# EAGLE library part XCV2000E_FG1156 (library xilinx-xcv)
xcv2000e_fg1156 edit this description Auto generated by make-symbol-device-package-bsdl.ulp Rev. 26 Source: xcv2000e_fg1156.bsd
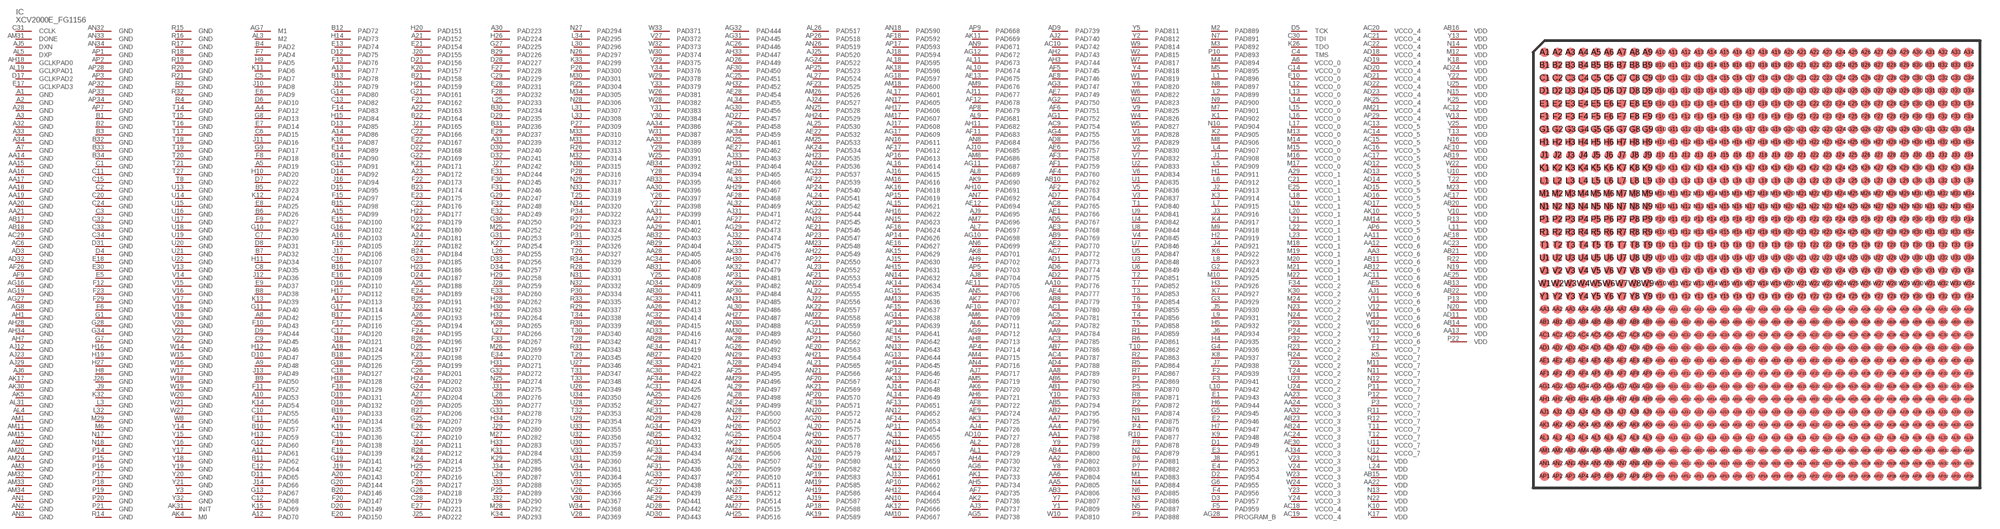
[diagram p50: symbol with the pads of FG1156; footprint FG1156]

Designator prefix IC

## XCV2000E_FG1156 (OC_FARNELL: unknown; OC_NEWARK: unknown)  [FG1156]
A1  GND  pwr
A2  GND  pwr
A3  GND  pwr
A4  PAD12
A5  PAD19
A6  VCCO_0  pwr
A7  GND  pwr
A8  PAD42
A9  PAD48
A10  PAD53
A11  PAD61
A12  PAD70
A13  PAD77
A14  PAD86
A15  PAD99
A16  PAD103
A17  PAD113
A18  PAD124
A19  PAD134
A20  PAD143
A21  PAD152
A22  PAD163
A23  PAD172
A24  PAD181
A25  PAD188
A26  PAD193
A27  PAD204
A28  GND  pwr
A29  VCCO_1  pwr
A30  PAD223
A31  PAD239
A32  GND  pwr
A33  GND  pwr
A34  GND  pwr
AA1  PAD798
AA2  PAD802
AA3  VCCO_6  pwr
AA4  PAD797
AA5  PAD805
AA6  PAD804
AA7  PAD796
AA8  PAD789
AA9  PAD784
AA10  PAD776
AA11  VCCO_6  pwr
AA12  VCCO_6  pwr
AA13  VDD  pwr
AA14  GND  pwr
AA15  GND  pwr
AA16  GND  pwr
AA17  GND  pwr
AA18  GND  pwr
AA19  GND  pwr
AA20  GND  pwr
AA21  GND  pwr
AA22  VDD  pwr
AA23  VCCO_3  pwr
AA24  VCCO_3  pwr
AA25  PAD426
AA26  PAD413
AA27  PAD401
AA28  PAD405
AA29  PAD402
AA30  PAD396
AA31  PAD399
AA32  VCCO_3  pwr
AA33  PAD389
AA34  PAD386
AB1  PAD792
AB2  PAD795
AB3  PAD806
AB4  PAD800
AB5  PAD794
AB6  PAD790
AB7  PAD786
AB8  PAD779
AB9  PAD769
AB10  PAD762
AB11  VCCO_6  pwr
AB12  VCCO_6  pwr
AB13  VDD  pwr
AB14  VDD  pwr
AB15  VDD  pwr
AB16  VDD  pwr
AB17  GND  pwr
AB18  GND  pwr
AB19  VDD  pwr
AB20  VDD  pwr
AB21  VDD  pwr
AB22  VDD  pwr
AB23  VCCO_3  pwr
AB24  VCCO_3  pwr
AB25  PAD432
AB26  PAD415
AB27  PAD420
AB28  PAD417
AB29  PAD404
AB30  PAD411
AB31  PAD407
AB32  PAD403
AB33  PAD395
AB34  PAD392
AC1  PAD780
AC2  PAD782
AC3  PAD785
AC4  PAD787
AC5  PAD781
AC6  GND  pwr
AC7  PAD772
AC8  PAD765
AC9  PAD754
AC10  PAD742
AC11  VCCO_6  pwr
AC12  VDD  pwr
AC13  VCCO_5  pwr
AC14  VCCO_5  pwr
AC15  VCCO_5  pwr
AC16  VCCO_5  pwr
AC17  VCCO_5  pwr
AC18  VCCO_4  pwr
AC19  VCCO_4  pwr
AC20  VCCO_4  pwr
AC21  VCCO_4  pwr
AC22  VCCO_4  pwr
AC23  VDD  pwr
AC24  VCCO_3  pwr
AC25  PAD451
AC26  PAD446
AC27  PAD438
AC28  PAD435
AC29  GND  pwr
AC30  PAD422
AC31  PAD425
AC32  PAD414
AC33  PAD412
AC34  PAD406
AD1  PAD773
AD2  PAD775
AD3  GND  pwr
AD4  PAD788
AD5  PAD767
AD6  PAD774
AD7  PAD764
AD8  PAD756
AD9  PAD739
AD10  PAD727
AD11  VDD  pwr
AD12  VCCO_5  pwr
AD13  VCCO_5  pwr
AD14  VCCO_5  pwr
AD15  VCCO_5  pwr
AD16  VCCO_5  pwr
AD17  VCCO_5  pwr
AD18  VCCO_4  pwr
AD19  VCCO_4  pwr
AD20  VCCO_4  pwr
AD21  VCCO_4  pwr
AD22  VCCO_4  pwr
AD23  VCCO_4  pwr
AD24  VDD  pwr
AD25  PAD461
AD26  PAD449
AD27  PAD457
AD28  PAD442
AD29  PAD429
AD30  PAD443
AD31  PAD433
AD32  GND  pwr
AD33  PAD416
AD34  PAD409
AE1  PAD766
AE2  PAD770
AE3  PAD768
AE4  PAD777
AE5  VCCO_6  pwr
AE6  PAD757
AE7  PAD749
AE8  PAD746
AE9  PAD724
AE10  VDD  pwr
AE11  PAD705
AE12  PAD694
AE13  PAD675
AE14  PAD641
AE15  PAD642
AE16  PAD627
AE17  VDD  pwr
AE18  VDD  pwr
AE19  PAD571
AE20  PAD563
AE21  PAD546
AE22  PAD532
AE23  PAD514
AE24  PAD499
AE25  VDD  pwr
AE26  PAD465
AE27  PAD462
AE28  PAD454
AE29  PAD441
AE30  VCCO_3  pwr
AE31  PAD428
AE32  PAD427
AE33  PAD421
AE34  PAD419
AF1  PAD759
AF2  PAD763
AF3  PAD758
AF4  PAD760
AF5  PAD745
AF6  PAD751
AF7  PAD735
AF8  PAD722
AF9  GND  pwr
AF10  PAD708
AF11  PAD683
AF12  PAD678
AF13  PAD651
AF14  PAD653
AF15  PAD637
AF16  PAD624
AF17  PAD612
AF18  PAD592
AF19  PAD582
AF20  PAD567
AF21  PAD553
AF22  PAD539
AF23  PAD525
AF24  PAD507
AF25  PAD495
AF26  GND  pwr
AF27  PAD472
AF28  PAD468
AF29  PAD458
AF30  PAD450
AF31  PAD436
AF32  PAD439
AF33  PAD434
AF34  PAD424
AG1  PAD752
AG2  PAD750
AG3  PAD747
AG4  PAD755
AG5  PAD738
AG6  PAD732
AG7  M1  in
AG8  GND  pwr
AG9  PAD712
AG10  PAD698
AG11  PAD687
AG12  PAD672
AG13  PAD644
AG14  PAD638
AG15  PAD635
AG16  GND  pwr
AG17  PAD609
AG18  PAD597
AG19  GND  pwr
AG20  PAD574
AG21  PAD559
AG22  PAD544
AG23  PAD537
AG24  PAD522
AG25  PAD504
AG26  PAD492
AG27  GND  pwr
AG28  PROGRAM_B  in
AG29  PAD473
AG30  PAD456
AG31  PAD445
AG32  PAD444
AG33  PAD437
AG34  PAD431
AH1  GND  pwr
AH2  PAD743
AH3  PAD744
AH4  PAD730
AH5  PAD734
AH6  PAD721
AH7  GND  pwr
AH8  PAD713
AH9  PAD702
AH10  PAD691
AH11  PAD682
AH12  PAD664
AH13  PAD657
AH14  PAD645
AH15  PAD631
AH16  PAD622
AH17  PAD606
AH18  GCLKPAD0  in
AH19  PAD586
AH20  PAD577
AH21  PAD564
AH22  PAD549
AH23  PAD535
AH24  PAD529
AH25  PAD516
AH26  PAD503
AH27  PAD487
AH28  GND  pwr
AH29  PAD467
AH30  PAD477
AH31  PAD464
AH32  PAD452
AH33  PAD447
AH34  GND  pwr
AJ1  VCCO_6  pwr
AJ2  PAD740
AJ3  PAD737
AJ4  PAD726
AJ5  DXN  pas
AJ6  GND  pwr
AJ7  PAD717
AJ8  PAD704
AJ9  PAD695
AJ10  PAD685
AJ11  PAD677
AJ12  GND  pwr
AJ13  PAD661
AJ14  PAD648
AJ15  PAD630
AJ16  PAD615
AJ17  PAD608
AJ18  PAD594
AJ19  PAD587
AJ20  PAD580
AJ21  PAD560
AJ22  PAD556
AJ23  GND  pwr
AJ24  PAD527
AJ25  PAD520
AJ26  PAD509
AJ27  PAD502
AJ28  PAD494
AJ29  GND  pwr
AJ30  PAD475
AJ31  PAD471
AJ32  PAD474
AJ33  PAD463
AJ34  VCCO_3  pwr
AK1  PAD733
AK2  PAD736
AK3  PAD725
AK4  M0  in
AK5  GND  pwr
AK6  PAD720
AK7  PAD707
AK8  PAD701
AK9  PAD690
AK10  VCCO_5  pwr
AK11  PAD669
AK12  PAD666
AK13  PAD647
AK14  PAD634
AK15  PAD629
AK16  PAD618
AK17  GND  pwr
AK18  PAD596
AK19  PAD589
AK20  PAD578
AK21  PAD569
AK22  PAD557
AK23  PAD542
AK24  PAD534
AK25  VCCO_4  pwr
AK26  PAD511
AK27  PAD505
AK28  PAD490
AK29  PAD482
AK30  GND  pwr
AK31  INIT
AK32  PAD479
AK33  PAD476
AK34  PAD459
AL1  PAD729
AL2  PAD728
AL3  M2  in
AL4  GND  pwr
AL5  DXP  pas
AL6  PAD711
AL7  PAD697
AL8  PAD689
AL9  PAD681
AL10  PAD674
AL11  PAD673
AL12  PAD660
AL13  PAD655
AL14  PAD649
AL15  PAD621
AL16  PAD614
AL17  PAD601
AL18  PAD595
AL19  GCLKPAD1  in
AL20  PAD575
AL21  PAD565
AL22  PAD555
AL23  PAD552
AL24  PAD541
AL25  PAD530
AL26  PAD517
AL27  PAD524
AL28  PAD498
AL29  PAD497
AL30  PAD486
AL31  GND  pwr
AL32  PAD469
AL33  PAD466
AL34  PAD455
AM1  GND  pwr
AM2  GND  pwr
AM3  GND  pwr
AM4  PAD715
AM5  PAD719
AM6  PAD709
AM7  PAD696
AM8  PAD686
AM9  PAD676
AM10  PAD667
AM11  GND  pwr
AM12  PAD659
AM13  PAD636
AM14  VCCO_5  pwr
AM15  GND  pwr
AM16  PAD616
AM17  PAD607
AM18  PAD600
AM19  PAD585
AM20  GND  pwr
AM21  VCCO_4  pwr
AM22  PAD558
AM23  PAD548
AM24  GND  pwr
AM25  PAD533
AM26  PAD526
AM27  PAD515
AM28  PAD506
AM29  PAD496
AM30  PAD489
AM31  DONE
AM32  GND  pwr
AM33  GND  pwr
AM34  GND  pwr
AN1  GND  pwr
AN2  GND  pwr
AN3  GND  pwr
AN4  PAD716
AN5  PAD706
AN6  PAD699
AN7  PAD692
AN8  PAD684
AN9  PAD671
AN10  PAD665
AN11  PAD656
AN12  PAD652
AN13  PAD643
AN14  PAD632
AN15  PAD623
AN16  PAD611
AN17  PAD605
AN18  PAD590
AN19  PAD579
AN20  PAD572
AN21  PAD566
AN22  PAD554
AN23  PAD545
AN24  PAD536
AN25  PAD528
AN26  PAD519
AN27  PAD512
AN28  PAD500
AN29  PAD493
AN30  PAD488
AN31  PAD485
AN32  GND  pwr
AN33  GND  pwr
AN34  GND  pwr
AP1  GND  pwr
AP2  GND  pwr
AP3  GND  pwr
AP4  PAD714
AP5  PAD703
AP6  VCCO_5  pwr
AP7  GND  pwr
AP8  PAD679
AP9  PAD668
AP10  PAD662
AP11  PAD654
AP12  PAD646
AP13  PAD639
AP14  PAD626
AP15  PAD619
AP16  PAD613
AP17  PAD593
AP18  PAD588
AP19  PAD583
AP20  PAD570
AP21  PAD562
AP22  PAD550
AP23  PAD547
AP24  PAD540
AP25  PAD523
AP26  PAD518
AP27  PAD510
AP28  GND  pwr
AP29  VCCO_4  pwr
AP30  PAD484
AP31  PAD481
AP32  GND  pwr
AP33  GND  pwr
AP34  GND  pwr
B1  GND  pwr
B2  GND  pwr
B3  GND  pwr
B4  PAD2
B5  PAD23
B6  PAD26
B7  PAD32
B8  PAD38
B9  PAD50
B10  PAD57
B11  PAD62
B12  PAD72
B13  PAD78
B14  PAD90
B15  PAD98
B16  PAD108
B17  PAD115
B18  PAD125
B19  PAD133
B20  PAD146
B21  PAD158
B22  PAD164
B23  PAD174
B24  PAD184
B25  PAD191
B26  PAD196
B27  PAD206
B28  PAD212
B29  PAD226
B30  PAD234
B31  PAD236
B32  GND  pwr
B33  GND  pwr
B34  GND  pwr
C1  GND  pwr
C2  GND  pwr
C3  GND  pwr
C4  TMS  in
C5  PAD7
C6  PAD15
C7  PAD30
C8  PAD35
C9  PAD45
C10  PAD55
C11  GND  pwr
C12  PAD68
C13  PAD82
C14  VCCO_0  pwr
C15  GND  pwr
C16  PAD107
C17  PAD120
C18  PAD127
C19  PAD136
C20  GND  pwr
C21  VCCO_1  pwr
C22  PAD166
C23  PAD176
C24  GND  pwr
C25  PAD194
C26  PAD201
C27  PAD210
C28  PAD219
C29  PAD229
C30  TDI  in
C31  CCLK
C32  GND  pwr
C33  GND  pwr
C34  GND  pwr
D1  PAD949
D2  PAD954
D3  PAD957
D4  GND  pwr
D5  TCK  in
D6  PAD10
D7  PAD22
D8  PAD31
D9  PAD44
D10  PAD47
D11  PAD65
D12  PAD75
D13  PAD85
D14  PAD92
D15  PAD95
D16  PAD110
D17  GCLKPAD2  in
D18  PAD132
D19  PAD131
D20  PAD149
D21  PAD156
D22  PAD168
D23  PAD179
D24  PAD187
D25  PAD197
D26  PAD205
D27  PAD216
D28  PAD227
D29  PAD235
D30  PAD240
D31  GND  pwr
D32  PAD241
D33  PAD256
D34  PAD257
E1  PAD943
E2  PAD946
E3  PAD951
E4  PAD953
E5  GND  pwr
E6  PAD9
E7  PAD14
E8  PAD25
E9  PAD37
E10  VCCO_0  pwr
E11  PAD56
E12  PAD64
E13  PAD74
E14  PAD89
E15  PAD100
E16  PAD109
E17  GCLKPAD3  in
E18  GND  pwr
E19  PAD139
E20  PAD150
E21  PAD154
E22  PAD167
E23  PAD175
E24  PAD189
E25  VCCO_1  pwr
E26  PAD209
E27  PAD221
E28  PAD231
E29  PAD237
E30  GND  pwr
E31  PAD244
E32  PAD249
E33  PAD260
E34  PAD270
F1  VCCO_7  pwr
F2  PAD939
F3  PAD941
F4  PAD956
F5  PAD959
F6  GND  pwr
F7  PAD4
F8  PAD18
F9  PAD27
F10  PAD43
F11  PAD52
F12  GND  pwr
F13  PAD76
F14  PAD83
F15  PAD97
F16  PAD105
F17  PAD116
F18  PAD129
F19  PAD138
F20  PAD147
F21  PAD162
F22  PAD173
F23  GND  pwr
F24  PAD195
F25  PAD199
F26  PAD217
F27  PAD228
F28  PAD232
F29  GND  pwr
F30  PAD245
F31  PAD246
F32  PAD248
F33  PAD267
F34  VCCO_2  pwr
G1  GND  pwr
G2  PAD924
G3  PAD929
G4  PAD936
G5  PAD945
G6  PAD955
G7  GND  pwr
G8  PAD13
G9  PAD17
G10  PAD29
G11  PAD40
G12  PAD60
G13  PAD67
G14  PAD80
G15  PAD91
G16  PAD102
G17  PAD114
G18  PAD126
G19  PAD141
G20  PAD144
G21  PAD161
G22  PAD169
G23  PAD185
G24  PAD203
G25  PAD207
G26  PAD218
G27  PAD225
G28  GND  pwr
G29  PAD247
G30  PAD250
G31  PAD253
G32  PAD272
G33  PAD278
G34  GND  pwr
H1  PAD911
H2  PAD919
H3  PAD926
H4  PAD935
H5  PAD932
H6  PAD944
H7  PAD947
H8  GND  pwr
H9  PAD5
H10  PAD20
H11  PAD34
H12  PAD46
H13  PAD59
H14  PAD73
H15  PAD84
H16  GND  pwr
H17  PAD112
H18  PAD128
H19  GND  pwr
H20  PAD151
H21  PAD159
H22  PAD177
H23  PAD186
H24  PAD202
H25  PAD215
H26  PAD224
H27  GND  pwr
H28  PAD262
H29  PAD258
H30  PAD263
H31  PAD271
H32  PAD264
H33  PAD283
H34  PAD279
J1  PAD908
J2  PAD913
J3  PAD916
J4  PAD921
J5  PAD930
J6  PAD934
J7  PAD938
J8  PAD952
J9  GND  pwr
J10  PAD8
J11  PAD16
J12  PAD36
J13  PAD49
J14  PAD66
J15  PAD79
J16  PAD94
J17  PAD106
J18  PAD121
J19  PAD142
J20  PAD155
J21  PAD165
J22  PAD182
J23  PAD192
J24  PAD211
J25  PAD222
J26  GND  pwr
J27  PAD242
J28  PAD259
J29  PAD280
J30  PAD277
J31  PAD275
J32  PAD290
J33  PAD288
J34  PAD286
K1  PAD902
K2  PAD905
K3  PAD914
K4  PAD917
K5  VCCO_7  pwr
K6  PAD922
K7  PAD927
K8  PAD937
K9  PAD948
K10  VDD  pwr
K11  PAD6
K12  PAD24
K13  PAD39
K14  PAD54
K15  PAD69
K16  PAD87
K17  VDD  pwr
K18  VDD  pwr
K19  PAD135
K20  PAD157
K21  PAD171
K22  PAD180
K23  PAD198
K24  PAD214
K25  VDD  pwr
K26  TDO  out
K27  PAD254
K28  PAD265
K29  PAD285
K30  VCCO_2  pwr
K31  PAD284
K32  GND  pwr
K33  PAD299
K34  PAD293
L1  PAD896
L2  PAD899
L3  GND  pwr
L4  PAD907
L5  PAD909
L6  PAD912
L7  PAD915
L8  PAD923
L9  PAD931
L10  PAD942
L11  VDD  pwr
L12  VCCO_0  pwr
L13  VCCO_0  pwr
L14  VCCO_0  pwr
L15  VCCO_0  pwr
L16  VCCO_0  pwr
L17  VCCO_0  pwr
L18  VCCO_1  pwr
L19  VCCO_1  pwr
L20  VCCO_1  pwr
L21  VCCO_1  pwr
L22  VCCO_1  pwr
L23  VCCO_1  pwr
L24  VDD  pwr
L25  PAD233
L26  PAD255
L27  PAD266
L28  PAD276
L29  PAD287
L30  PAD296
L31  PAD307
L32  GND  pwr
L33  PAD308
L34  PAD295
M1  PAD883
M2  PAD889
M3  PAD892
M4  PAD894
M5  PAD895
M6  GND  pwr
M7  PAD901
M8  PAD906
M9  PAD918
M10  PAD925
M11  VCCO_7  pwr
M12  VDD  pwr
M13  VCCO_0  pwr
M14  VCCO_0  pwr
M15  VCCO_0  pwr
M16  VCCO_0  pwr
M17  VCCO_0  pwr
M18  VCCO_1  pwr
M19  VCCO_1  pwr
M20  VCCO_1  pwr
M21  VCCO_1  pwr
M22  VCCO_1  pwr
M23  VDD  pwr
M24  VCCO_2  pwr
M25  PAD252
M26  PAD269
M27  PAD282
M28  PAD292
M29  GND  pwr
M30  PAD301
M31  PAD312
M32  PAD314
M33  PAD310
M34  PAD305
N1  PAD875
N2  PAD879
N3  PAD886
N4  PAD884
N5  PAD887
N6  PAD885
N7  PAD891
N8  PAD897
N9  PAD900
N10  PAD904
N11  VCCO_7  pwr
N12  VCCO_7  pwr
N13  VDD  pwr
N14  VDD  pwr
N15  VDD  pwr
N16  VDD  pwr
N17  GND  pwr
N18  GND  pwr
N19  VDD  pwr
N20  VDD  pwr
N21  VDD  pwr
N22  VDD  pwr
N23  VCCO_2  pwr
N24  VCCO_2  pwr
N25  PAD274
N26  PAD297
N27  PAD294
N28  PAD306
N29  PAD317
N30  PAD315
N31  PAD331
N32  PAD332
N33  PAD318
N34  PAD320
P1  PAD869
P2  PAD872
P3  VCCO_7  pwr
P4  PAD876
P5  PAD870
P6  PAD881
P7  PAD882
P8  PAD878
P9  PAD888
P10  PAD893
P11  VCCO_7  pwr
P12  VCCO_7  pwr
P13  VDD  pwr
P14  GND  pwr
P15  GND  pwr
P16  GND  pwr
P17  GND  pwr
P18  GND  pwr
P19  GND  pwr
P20  GND  pwr
P21  GND  pwr
P22  VDD  pwr
P23  VCCO_2  pwr
P24  VCCO_2  pwr
P25  PAD289
P26  PAD300
P27  PAD309
P28  PAD316
P29  PAD324
P30  PAD334
P31  PAD325
P32  VCCO_2  pwr
P33  PAD326
P34  PAD322
R1  PAD859
R2  PAD863
R3  GND  pwr
R4  GND  pwr
R5  PAD864
R6  PAD861
R7  PAD867
R8  PAD871
R9  PAD874
R10  PAD877
R11  VCCO_7  pwr
R12  VCCO_7  pwr
R13  VDD  pwr
R14  GND  pwr
R15  GND  pwr
R16  GND  pwr
R17  GND  pwr
R18  GND  pwr
R19  GND  pwr
R20  GND  pwr
R21  GND  pwr
R22  VDD  pwr
R23  VCCO_2  pwr
R24  VCCO_2  pwr
R25  PAD304
R26  PAD313
R27  PAD323
R28  PAD330
R29  PAD337
R30  PAD339
R31  PAD343
R32  GND  pwr
R33  PAD335
R34  PAD329
T1  PAD840
T2  PAD851
T3  PAD853
T4  PAD856
T5  PAD858
T6  PAD854
T7  PAD852
T8  GND  pwr
T9  PAD855
T10  PAD862
T11  VCCO_7  pwr
T12  VCCO_7  pwr
T13  VDD  pwr
T14  GND  pwr
T15  GND  pwr
T16  GND  pwr
T17  GND  pwr
T18  GND  pwr
T19  GND  pwr
T20  GND  pwr
T21  GND  pwr
T22  VDD  pwr
T23  VCCO_2  pwr
T24  VCCO_2  pwr
T25  PAD319
T26  PAD327
T27  GND  pwr
T28  PAD342
T29  PAD345
T30  PAD340
T31  PAD347
T32  PAD353
T33  PAD348
T34  PAD338
U1  PAD835
U2  PAD833
U3  PAD848
U4  PAD842
U5  PAD847
U6  PAD849
U7  PAD846
U8  PAD844
U9  PAD841
U10  VDD  pwr
U11  VCCO_7  pwr
U12  VCCO_7  pwr
U13  GND  pwr
U14  GND  pwr
U15  GND  pwr
U16  GND  pwr
U17  GND  pwr
U18  GND  pwr
U19  GND  pwr
U20  GND  pwr
U21  GND  pwr
U22  GND  pwr
U23  VCCO_2  pwr
U24  VCCO_2  pwr
U25  VDD  pwr
U26  PAD349
U27  PAD346
U28  PAD352
U29  PAD354
U30  PAD357
U31  PAD360
U32  PAD356
U33  PAD355
U34  PAD350
V1  PAD828
V2  PAD830
V3  PAD837
V4  PAD845
V5  PAD836
V6  PAD834
V7  PAD832
V8  PAD829
V9  PAD825
V10  VDD  pwr
V11  VCCO_6  pwr
V12  VCCO_6  pwr
V13  GND  pwr
V14  GND  pwr
V15  GND  pwr
V16  GND  pwr
V17  GND  pwr
V18  GND  pwr
V19  GND  pwr
V20  GND  pwr
V21  GND  pwr
V22  GND  pwr
V23  VCCO_3  pwr
V24  VCCO_3  pwr
V25  VDD  pwr
V26  PAD366
V27  PAD372
V28  PAD369
V29  PAD375
V30  PAD367
V31  PAD364
V32  PAD365
V33  PAD359
V34  PAD361
W1  PAD819
W2  PAD815
W3  PAD823
W4  PAD826
W5  PAD827
W6  PAD822
W7  PAD817
W8  GND  pwr
W9  PAD814
W10  PAD810
W11  VCCO_6  pwr
W12  VCCO_6  pwr
W13  VDD  pwr
W14  GND  pwr
W15  GND  pwr
W16  GND  pwr
W17  GND  pwr
W18  GND  pwr
W19  GND  pwr
W20  GND  pwr
W21  GND  pwr
W22  VDD  pwr
W23  VCCO_3  pwr
W24  VCCO_3  pwr
W25  PAD391
W26  PAD381
W27  GND  pwr
W28  PAD382
W29  PAD378
W30  PAD374
W31  PAD387
W32  PAD373
W33  PAD371
W34  PAD368
Y1  PAD809
Y2  PAD812
Y3  GND  pwr
Y4  PAD818
Y5  PAD811
Y6  PAD820
Y7  PAD807
Y8  PAD803
Y9  PAD799
Y10  PAD793
Y11  VCCO_6  pwr
Y12  VCCO_6  pwr
Y13  VDD  pwr
Y14  GND  pwr
Y15  GND  pwr
Y16  GND  pwr
Y17  GND  pwr
Y18  GND  pwr
Y19  GND  pwr
Y20  GND  pwr
Y21  GND  pwr
Y22  VDD  pwr
Y23  VCCO_3  pwr
Y24  VCCO_3  pwr
Y25  PAD408
Y26  PAD397
Y27  PAD398
Y28  PAD394
Y29  PAD390
Y30  PAD384
Y31  PAD383
Y32  GND  pwr
Y33  PAD379
Y34  PAD376

## Footprint FG1156 (pad centres in mm)
xcv1000e_fg1156_1532 edit this description Auto generated by make-symbol-device-package-bsdl.ulp Rev. 26 Source: xcv1000e_fg1156_1532.bsd
smd 0.7 x 0.7: A1 -16.5,16.5; A2 -15.5,16.5; A3 -14.5,16.5; A4 -13.5,16.5; A5 -12.5,16.5; A6 -11.5,16.5; A7 -10.5,16.5; A8 -9.5,16.5; A9 -8.5,16.5; A10 -7.5,16.5; A11 -6.5,16.5; A12 -5.5,16.5; A13 -4.5,16.5; A14 -3.5,16.5; A15 -2.5,16.5; A16 -1.5,16.5; A17 -0.5,16.5; A18 0.5,16.5; A19 1.5,16.5; A20 2.5,16.5; A21 3.5,16.5; A22 4.5,16.5; A23 5.5,16.5; A24 6.5,16.5; A25 7.5,16.5; A26 8.5,16.5; A27 9.5,16.5; A28 10.5,16.5; A29 11.5,16.5; A30 12.5,16.5; A31 13.5,16.5; A32 14.5,16.5; A33 15.5,16.5; A34 16.5,16.5; AA1 -16.5,-3.5; AA2 -15.5,-3.5; AA3 -14.5,-3.5; AA4 -13.5,-3.5; AA5 -12.5,-3.5; AA6 -11.5,-3.5; AA7 -10.5,-3.5; AA8 -9.5,-3.5; AA9 -8.5,-3.5; AA10 -7.5,-3.5; AA11 -6.5,-3.5; AA12 -5.5,-3.5; AA13 -4.5,-3.5; AA14 -3.5,-3.5; AA15 -2.5,-3.5; AA16 -1.5,-3.5; AA17 -0.5,-3.5; AA18 0.5,-3.5; AA19 1.5,-3.5; AA20 2.5,-3.5; AA21 3.5,-3.5; AA22 4.5,-3.5; AA23 5.5,-3.5; AA24 6.5,-3.5; AA25 7.5,-3.5; AA26 8.5,-3.5; AA27 9.5,-3.5; AA28 10.5,-3.5; AA29 11.5,-3.5; AA30 12.5,-3.5; AA31 13.5,-3.5; AA32 14.5,-3.5; AA33 15.5,-3.5; AA34 16.5,-3.5; AB1 -16.5,-4.5; AB2 -15.5,-4.5; AB3 -14.5,-4.5; AB4 -13.5,-4.5; AB5 -12.5,-4.5; AB6 -11.5,-4.5; AB7 -10.5,-4.5; AB8 -9.5,-4.5; AB9 -8.5,-4.5; AB10 -7.5,-4.5; AB11 -6.5,-4.5; AB12 -5.5,-4.5; AB13 -4.5,-4.5; AB14 -3.5,-4.5; AB15 -2.5,-4.5; AB16 -1.5,-4.5; AB17 -0.5,-4.5; AB18 0.5,-4.5; AB19 1.5,-4.5; AB20 2.5,-4.5; AB21 3.5,-4.5; AB22 4.5,-4.5; AB23 5.5,-4.5; AB24 6.5,-4.5; AB25 7.5,-4.5; AB26 8.5,-4.5; AB27 9.5,-4.5; AB28 10.5,-4.5; AB29 11.5,-4.5; AB30 12.5,-4.5; AB31 13.5,-4.5; AB32 14.5,-4.5; AB33 15.5,-4.5; AB34 16.5,-4.5; AC1 -16.5,-5.5; AC2 -15.5,-5.5; AC3 -14.5,-5.5; AC4 -13.5,-5.5; AC5 -12.5,-5.5; AC6 -11.5,-5.5; AC7 -10.5,-5.5; AC8 -9.5,-5.5; AC9 -8.5,-5.5; AC10 -7.5,-5.5; AC11 -6.5,-5.5; AC12 -5.5,-5.5; AC13 -4.5,-5.5; AC14 -3.5,-5.5; AC15 -2.5,-5.5; AC16 -1.5,-5.5; AC17 -0.5,-5.5; AC18 0.5,-5.5; AC19 1.5,-5.5; AC20 2.5,-5.5; AC21 3.5,-5.5; AC22 4.5,-5.5; AC23 5.5,-5.5; AC24 6.5,-5.5; AC25 7.5,-5.5; AC26 8.5,-5.5; AC27 9.5,-5.5; AC28 10.5,-5.5; AC29 11.5,-5.5; AC30 12.5,-5.5; AC31 13.5,-5.5; AC32 14.5,-5.5; AC33 15.5,-5.5; AC34 16.5,-5.5; AD1 -16.5,-6.5; AD2 -15.5,-6.5; AD3 -14.5,-6.5; AD4 -13.5,-6.5; AD5 -12.5,-6.5; AD6 -11.5,-6.5; AD7 -10.5,-6.5; AD8 -9.5,-6.5; AD9 -8.5,-6.5; AD10 -7.5,-6.5; AD11 -6.5,-6.5; AD12 -5.5,-6.5; AD13 -4.5,-6.5; AD14 -3.5,-6.5; AD15 -2.5,-6.5; AD16 -1.5,-6.5; AD17 -0.5,-6.5; AD18 0.5,-6.5; AD19 1.5,-6.5; AD20 2.5,-6.5; AD21 3.5,-6.5; AD22 4.5,-6.5; AD23 5.5,-6.5; AD24 6.5,-6.5; AD25 7.5,-6.5; AD26 8.5,-6.5; AD27 9.5,-6.5; AD28 10.5,-6.5; AD29 11.5,-6.5; AD30 12.5,-6.5; AD31 13.5,-6.5; AD32 14.5,-6.5; AD33 15.5,-6.5; AD34 16.5,-6.5; AE1 -16.5,-7.5; AE2 -15.5,-7.5; AE3 -14.5,-7.5; AE4 -13.5,-7.5; AE5 -12.5,-7.5; AE6 -11.5,-7.5; AE7 -10.5,-7.5; AE8 -9.5,-7.5; AE9 -8.5,-7.5; AE10 -7.5,-7.5; AE11 -6.5,-7.5; AE12 -5.5,-7.5; AE13 -4.5,-7.5; AE14 -3.5,-7.5; AE15 -2.5,-7.5; AE16 -1.5,-7.5; AE17 -0.5,-7.5; AE18 0.5,-7.5; AE19 1.5,-7.5; AE20 2.5,-7.5; AE21 3.5,-7.5; AE22 4.5,-7.5; AE23 5.5,-7.5; AE24 6.5,-7.5; AE25 7.5,-7.5; AE26 8.5,-7.5; AE27 9.5,-7.5; AE28 10.5,-7.5; AE29 11.5,-7.5; AE30 12.5,-7.5; AE31 13.5,-7.5; AE32 14.5,-7.5; AE33 15.5,-7.5; AE34 16.5,-7.5; AF1 -16.5,-8.5; AF2 -15.5,-8.5; AF3 -14.5,-8.5; AF4 -13.5,-8.5; AF5 -12.5,-8.5; AF6 -11.5,-8.5; AF7 -10.5,-8.5; AF8 -9.5,-8.5; AF9 -8.5,-8.5; AF10 -7.5,-8.5; AF11 -6.5,-8.5; AF12 -5.5,-8.5; AF13 -4.5,-8.5; AF14 -3.5,-8.5; AF15 -2.5,-8.5; AF16 -1.5,-8.5; AF17 -0.5,-8.5; AF18 0.5,-8.5; AF19 1.5,-8.5; AF20 2.5,-8.5; AF21 3.5,-8.5; AF22 4.5,-8.5; AF23 5.5,-8.5; AF24 6.5,-8.5; AF25 7.5,-8.5; AF26 8.5,-8.5; AF27 9.5,-8.5; AF28 10.5,-8.5; AF29 11.5,-8.5; AF30 12.5,-8.5; AF31 13.5,-8.5; AF32 14.5,-8.5; AF33 15.5,-8.5; AF34 16.5,-8.5; AG1 -16.5,-9.5; AG2 -15.5,-9.5; AG3 -14.5,-9.5; AG4 -13.5,-9.5; AG5 -12.5,-9.5; AG6 -11.5,-9.5; AG7 -10.5,-9.5; AG8 -9.5,-9.5; AG9 -8.5,-9.5; AG10 -7.5,-9.5; AG11 -6.5,-9.5; AG12 -5.5,-9.5; AG13 -4.5,-9.5; AG14 -3.5,-9.5; AG15 -2.5,-9.5; AG16 -1.5,-9.5; AG17 -0.5,-9.5; AG18 0.5,-9.5; AG19 1.5,-9.5; AG20 2.5,-9.5; AG21 3.5,-9.5; AG22 4.5,-9.5; AG23 5.5,-9.5; AG24 6.5,-9.5; AG25 7.5,-9.5; AG26 8.5,-9.5; AG27 9.5,-9.5; AG28 10.5,-9.5; AG29 11.5,-9.5; AG30 12.5,-9.5; AG31 13.5,-9.5; AG32 14.5,-9.5; AG33 15.5,-9.5; AG34 16.5,-9.5; AH1 -16.5,-10.5; AH2 -15.5,-10.5; AH3 -14.5,-10.5; AH4 -13.5,-10.5; AH5 -12.5,-10.5; AH6 -11.5,-10.5; AH7 -10.5,-10.5; AH8 -9.5,-10.5; AH9 -8.5,-10.5; AH10 -7.5,-10.5; AH11 -6.5,-10.5; AH12 -5.5,-10.5; AH13 -4.5,-10.5; AH14 -3.5,-10.5; AH15 -2.5,-10.5; AH16 -1.5,-10.5; AH17 -0.5,-10.5; AH18 0.5,-10.5; AH19 1.5,-10.5; AH20 2.5,-10.5; AH21 3.5,-10.5; AH22 4.5,-10.5; AH23 5.5,-10.5; AH24 6.5,-10.5; AH25 7.5,-10.5; AH26 8.5,-10.5; AH27 9.5,-10.5; AH28 10.5,-10.5; AH29 11.5,-10.5; AH30 12.5,-10.5; AH31 13.5,-10.5; AH32 14.5,-10.5; AH33 15.5,-10.5; AH34 16.5,-10.5; AJ1 -16.5,-11.5; AJ2 -15.5,-11.5; AJ3 -14.5,-11.5; AJ4 -13.5,-11.5; AJ5 -12.5,-11.5; AJ6 -11.5,-11.5; AJ7 -10.5,-11.5; AJ8 -9.5,-11.5; AJ9 -8.5,-11.5; AJ10 -7.5,-11.5; AJ11 -6.5,-11.5; AJ12 -5.5,-11.5; AJ13 -4.5,-11.5; AJ14 -3.5,-11.5; AJ15 -2.5,-11.5; AJ16 -1.5,-11.5; AJ17 -0.5,-11.5; AJ18 0.5,-11.5; AJ19 1.5,-11.5; AJ20 2.5,-11.5; AJ21 3.5,-11.5; AJ22 4.5,-11.5; AJ23 5.5,-11.5; AJ24 6.5,-11.5; AJ25 7.5,-11.5; AJ26 8.5,-11.5; AJ27 9.5,-11.5; AJ28 10.5,-11.5; AJ29 11.5,-11.5; AJ30 12.5,-11.5; AJ31 13.5,-11.5; AJ32 14.5,-11.5; AJ33 15.5,-11.5; AJ34 16.5,-11.5; AK1 -16.5,-12.5; AK2 -15.5,-12.5; AK3 -14.5,-12.5; AK4 -13.5,-12.5; AK5 -12.5,-12.5; AK6 -11.5,-12.5; AK7 -10.5,-12.5; AK8 -9.5,-12.5; AK9 -8.5,-12.5; AK10 -7.5,-12.5; AK11 -6.5,-12.5; AK12 -5.5,-12.5; AK13 -4.5,-12.5; AK14 -3.5,-12.5; AK15 -2.5,-12.5; AK16 -1.5,-12.5; AK17 -0.5,-12.5; AK18 0.5,-12.5; AK19 1.5,-12.5; AK20 2.5,-12.5; AK21 3.5,-12.5; AK22 4.5,-12.5; AK23 5.5,-12.5; AK24 6.5,-12.5; AK25 7.5,-12.5; AK26 8.5,-12.5; AK27 9.5,-12.5; AK28 10.5,-12.5; AK29 11.5,-12.5; AK30 12.5,-12.5; AK31 13.5,-12.5; AK32 14.5,-12.5; AK33 15.5,-12.5; AK34 16.5,-12.5; AL1 -16.5,-13.5; AL2 -15.5,-13.5; AL3 -14.5,-13.5; AL4 -13.5,-13.5; AL5 -12.5,-13.5; AL6 -11.5,-13.5; AL7 -10.5,-13.5; AL8 -9.5,-13.5; AL9 -8.5,-13.5; AL10 -7.5,-13.5; AL11 -6.5,-13.5; AL12 -5.5,-13.5; AL13 -4.5,-13.5; AL14 -3.5,-13.5; AL15 -2.5,-13.5; AL16 -1.5,-13.5; AL17 -0.5,-13.5; AL18 0.5,-13.5; AL19 1.5,-13.5; AL20 2.5,-13.5; AL21 3.5,-13.5; AL22 4.5,-13.5; AL23 5.5,-13.5; AL24 6.5,-13.5; AL25 7.5,-13.5; AL26 8.5,-13.5; AL27 9.5,-13.5; AL28 10.5,-13.5; AL29 11.5,-13.5; AL30 12.5,-13.5; AL31 13.5,-13.5; AL32 14.5,-13.5; AL33 15.5,-13.5; AL34 16.5,-13.5; AM1 -16.5,-14.5; AM2 -15.5,-14.5; AM3 -14.5,-14.5; AM4 -13.5,-14.5; AM5 -12.5,-14.5; AM6 -11.5,-14.5; AM7 -10.5,-14.5; AM8 -9.5,-14.5; AM9 -8.5,-14.5; AM10 -7.5,-14.5; AM11 -6.5,-14.5; AM12 -5.5,-14.5; AM13 -4.5,-14.5; AM14 -3.5,-14.5; AM15 -2.5,-14.5; AM16 -1.5,-14.5; AM17 -0.5,-14.5; AM18 0.5,-14.5; AM19 1.5,-14.5; AM20 2.5,-14.5; AM21 3.5,-14.5; AM22 4.5,-14.5; AM23 5.5,-14.5; AM24 6.5,-14.5; AM25 7.5,-14.5; AM26 8.5,-14.5; AM27 9.5,-14.5; AM28 10.5,-14.5; AM29 11.5,-14.5; AM30 12.5,-14.5; AM31 13.5,-14.5; AM32 14.5,-14.5; AM33 15.5,-14.5; AM34 16.5,-14.5; AN1 -16.5,-15.5; AN2 -15.5,-15.5; AN3 -14.5,-15.5; AN4 -13.5,-15.5; AN5 -12.5,-15.5; AN6 -11.5,-15.5; AN7 -10.5,-15.5; AN8 -9.5,-15.5; AN9 -8.5,-15.5; AN10 -7.5,-15.5; AN11 -6.5,-15.5; AN12 -5.5,-15.5; AN13 -4.5,-15.5; AN14 -3.5,-15.5; AN15 -2.5,-15.5; AN16 -1.5,-15.5; AN17 -0.5,-15.5; AN18 0.5,-15.5; AN19 1.5,-15.5; AN20 2.5,-15.5; AN21 3.5,-15.5; AN22 4.5,-15.5; AN23 5.5,-15.5; AN24 6.5,-15.5; AN25 7.5,-15.5; AN26 8.5,-15.5; AN27 9.5,-15.5; AN28 10.5,-15.5; AN29 11.5,-15.5; AN30 12.5,-15.5; AN31 13.5,-15.5; AN32 14.5,-15.5; AN33 15.5,-15.5; AN34 16.5,-15.5; AP1 -16.5,-16.5; AP2 -15.5,-16.5; AP3 -14.5,-16.5; AP4 -13.5,-16.5; AP5 -12.5,-16.5; AP6 -11.5,-16.5; AP7 -10.5,-16.5; AP8 -9.5,-16.5; AP9 -8.5,-16.5; AP10 -7.5,-16.5; AP11 -6.5,-16.5; AP12 -5.5,-16.5; AP13 -4.5,-16.5; AP14 -3.5,-16.5; AP15 -2.5,-16.5; AP16 -1.5,-16.5; AP17 -0.5,-16.5; AP18 0.5,-16.5; AP19 1.5,-16.5; AP20 2.5,-16.5; AP21 3.5,-16.5; AP22 4.5,-16.5; AP23 5.5,-16.5; AP24 6.5,-16.5; AP25 7.5,-16.5; AP26 8.5,-16.5; AP27 9.5,-16.5; AP28 10.5,-16.5; AP29 11.5,-16.5; AP30 12.5,-16.5; AP31 13.5,-16.5; AP32 14.5,-16.5; AP33 15.5,-16.5; AP34 16.5,-16.5; B1 -16.5,15.5; B2 -15.5,15.5; B3 -14.5,15.5; B4 -13.5,15.5; B5 -12.5,15.5; B6 -11.5,15.5; B7 -10.5,15.5; B8 -9.5,15.5; B9 -8.5,15.5; B10 -7.5,15.5; B11 -6.5,15.5; B12 -5.5,15.5; B13 -4.5,15.5; B14 -3.5,15.5; B15 -2.5,15.5; B16 -1.5,15.5; B17 -0.5,15.5; B18 0.5,15.5; B19 1.5,15.5; B20 2.5,15.5; B21 3.5,15.5; B22 4.5,15.5; B23 5.5,15.5; B24 6.5,15.5; B25 7.5,15.5; B26 8.5,15.5; B27 9.5,15.5; B28 10.5,15.5; B29 11.5,15.5; B30 12.5,15.5; B31 13.5,15.5; B32 14.5,15.5; B33 15.5,15.5; B34 16.5,15.5; C1 -16.5,14.5; C2 -15.5,14.5; C3 -14.5,14.5; C4 -13.5,14.5; C5 -12.5,14.5; C6 -11.5,14.5; C7 -10.5,14.5; C8 -9.5,14.5; C9 -8.5,14.5; C10 -7.5,14.5; C11 -6.5,14.5; C12 -5.5,14.5; C13 -4.5,14.5; C14 -3.5,14.5; C15 -2.5,14.5; C16 -1.5,14.5; C17 -0.5,14.5; C18 0.5,14.5; C19 1.5,14.5; C20 2.5,14.5; C21 3.5,14.5; C22 4.5,14.5; C23 5.5,14.5; C24 6.5,14.5; C25 7.5,14.5; C26 8.5,14.5; C27 9.5,14.5; C28 10.5,14.5; C29 11.5,14.5; C30 12.5,14.5; C31 13.5,14.5; C32 14.5,14.5; C33 15.5,14.5; C34 16.5,14.5; D1 -16.5,13.5; D2 -15.5,13.5; D3 -14.5,13.5; D4 -13.5,13.5; D5 -12.5,13.5; D6 -11.5,13.5; D7 -10.5,13.5; D8 -9.5,13.5; D9 -8.5,13.5; D10 -7.5,13.5; D11 -6.5,13.5; D12 -5.5,13.5; D13 -4.5,13.5; D14 -3.5,13.5; D15 -2.5,13.5; D16 -1.5,13.5; D17 -0.5,13.5; D18 0.5,13.5; D19 1.5,13.5; D20 2.5,13.5; D21 3.5,13.5; D22 4.5,13.5; D23 5.5,13.5; D24 6.5,13.5; D25 7.5,13.5; D26 8.5,13.5; D27 9.5,13.5; D28 10.5,13.5; D29 11.5,13.5; D30 12.5,13.5; D31 13.5,13.5; D32 14.5,13.5; D33 15.5,13.5; D34 16.5,13.5; E1 -16.5,12.5; E2 -15.5,12.5; E3 -14.5,12.5; E4 -13.5,12.5; E5 -12.5,12.5; E6 -11.5,12.5; E7 -10.5,12.5; E8 -9.5,12.5; E9 -8.5,12.5; E10 -7.5,12.5; E11 -6.5,12.5; E12 -5.5,12.5; E13 -4.5,12.5; E14 -3.5,12.5; E15 -2.5,12.5; E16 -1.5,12.5; E17 -0.5,12.5; E18 0.5,12.5; E19 1.5,12.5; E20 2.5,12.5; E21 3.5,12.5; E22 4.5,12.5; E23 5.5,12.5; E24 6.5,12.5; E25 7.5,12.5; E26 8.5,12.5; E27 9.5,12.5; E28 10.5,12.5; E29 11.5,12.5; E30 12.5,12.5; E31 13.5,12.5; E32 14.5,12.5; E33 15.5,12.5; E34 16.5,12.5; F1 -16.5,11.5; F2 -15.5,11.5; F3 -14.5,11.5; F4 -13.5,11.5; F5 -12.5,11.5; F6 -11.5,11.5; F7 -10.5,11.5; F8 -9.5,11.5; F9 -8.5,11.5; F10 -7.5,11.5; F11 -6.5,11.5; F12 -5.5,11.5; F13 -4.5,11.5; F14 -3.5,11.5; F15 -2.5,11.5; F16 -1.5,11.5; F17 -0.5,11.5; F18 0.5,11.5; F19 1.5,11.5; F20 2.5,11.5; F21 3.5,11.5; F22 4.5,11.5; F23 5.5,11.5; F24 6.5,11.5; F25 7.5,11.5; F26 8.5,11.5; F27 9.5,11.5; F28 10.5,11.5; F29 11.5,11.5; F30 12.5,11.5; F31 13.5,11.5; F32 14.5,11.5; F33 15.5,11.5; F34 16.5,11.5; G1 -16.5,10.5; G2 -15.5,10.5; G3 -14.5,10.5; G4 -13.5,10.5; G5 -12.5,10.5; G6 -11.5,10.5; G7 -10.5,10.5; G8 -9.5,10.5; G9 -8.5,10.5; G10 -7.5,10.5; G11 -6.5,10.5; G12 -5.5,10.5; G13 -4.5,10.5; G14 -3.5,10.5; G15 -2.5,10.5; G16 -1.5,10.5; G17 -0.5,10.5; G18 0.5,10.5; G19 1.5,10.5; G20 2.5,10.5; G21 3.5,10.5; G22 4.5,10.5; G23 5.5,10.5; G24 6.5,10.5; G25 7.5,10.5; G26 8.5,10.5; G27 9.5,10.5; G28 10.5,10.5; G29 11.5,10.5; G30 12.5,10.5; G31 13.5,10.5; G32 14.5,10.5; G33 15.5,10.5; G34 16.5,10.5; H1 -16.5,9.5; H2 -15.5,9.5; H3 -14.5,9.5; H4 -13.5,9.5; H5 -12.5,9.5; H6 -11.5,9.5; H7 -10.5,9.5; H8 -9.5,9.5; H9 -8.5,9.5; H10 -7.5,9.5; H11 -6.5,9.5; H12 -5.5,9.5; H13 -4.5,9.5; H14 -3.5,9.5; H15 -2.5,9.5; H16 -1.5,9.5; H17 -0.5,9.5; H18 0.5,9.5; H19 1.5,9.5; H20 2.5,9.5; H21 3.5,9.5; H22 4.5,9.5; H23 5.5,9.5; H24 6.5,9.5; H25 7.5,9.5; H26 8.5,9.5; H27 9.5,9.5; H28 10.5,9.5; H29 11.5,9.5; H30 12.5,9.5; H31 13.5,9.5; H32 14.5,9.5; H33 15.5,9.5; H34 16.5,9.5; J1 -16.5,8.5; J2 -15.5,8.5; J3 -14.5,8.5; J4 -13.5,8.5; J5 -12.5,8.5; J6 -11.5,8.5; J7 -10.5,8.5; J8 -9.5,8.5; J9 -8.5,8.5; J10 -7.5,8.5; J11 -6.5,8.5; J12 -5.5,8.5; J13 -4.5,8.5; J14 -3.5,8.5; J15 -2.5,8.5; J16 -1.5,8.5; J17 -0.5,8.5; J18 0.5,8.5; J19 1.5,8.5; J20 2.5,8.5; J21 3.5,8.5; J22 4.5,8.5; J23 5.5,8.5; J24 6.5,8.5; J25 7.5,8.5; J26 8.5,8.5; J27 9.5,8.5; J28 10.5,8.5; J29 11.5,8.5; J30 12.5,8.5; J31 13.5,8.5; J32 14.5,8.5; J33 15.5,8.5; J34 16.5,8.5; K1 -16.5,7.5; K2 -15.5,7.5; K3 -14.5,7.5; K4 -13.5,7.5; K5 -12.5,7.5; K6 -11.5,7.5; K7 -10.5,7.5; K8 -9.5,7.5; K9 -8.5,7.5; K10 -7.5,7.5; K11 -6.5,7.5; K12 -5.5,7.5; K13 -4.5,7.5; K14 -3.5,7.5; K15 -2.5,7.5; K16 -1.5,7.5; K17 -0.5,7.5; K18 0.5,7.5; K19 1.5,7.5; K20 2.5,7.5; K21 3.5,7.5; K22 4.5,7.5; K23 5.5,7.5; K24 6.5,7.5; K25 7.5,7.5; K26 8.5,7.5; K27 9.5,7.5; K28 10.5,7.5; K29 11.5,7.5; K30 12.5,7.5; K31 13.5,7.5; K32 14.5,7.5; K33 15.5,7.5; K34 16.5,7.5; L1 -16.5,6.5; L2 -15.5,6.5; L3 -14.5,6.5; L4 -13.5,6.5; L5 -12.5,6.5; L6 -11.5,6.5; L7 -10.5,6.5; L8 -9.5,6.5; L9 -8.5,6.5; L10 -7.5,6.5; L11 -6.5,6.5; L12 -5.5,6.5; L13 -4.5,6.5; L14 -3.5,6.5; L15 -2.5,6.5; L16 -1.5,6.5; L17 -0.5,6.5; L18 0.5,6.5; L19 1.5,6.5; L20 2.5,6.5; L21 3.5,6.5; L22 4.5,6.5; L23 5.5,6.5; L24 6.5,6.5; L25 7.5,6.5; L26 8.5,6.5; L27 9.5,6.5; L28 10.5,6.5; L29 11.5,6.5; L30 12.5,6.5; L31 13.5,6.5; L32 14.5,6.5; L33 15.5,6.5; L34 16.5,6.5; M1 -16.5,5.5; M2 -15.5,5.5; M3 -14.5,5.5; M4 -13.5,5.5; M5 -12.5,5.5; M6 -11.5,5.5; M7 -10.5,5.5; M8 -9.5,5.5; M9 -8.5,5.5; M10 -7.5,5.5; M11 -6.5,5.5; M12 -5.5,5.5; M13 -4.5,5.5; M14 -3.5,5.5; M15 -2.5,5.5; M16 -1.5,5.5; M17 -0.5,5.5; M18 0.5,5.5; M19 1.5,5.5; M20 2.5,5.5; M21 3.5,5.5; M22 4.5,5.5; M23 5.5,5.5; M24 6.5,5.5; M25 7.5,5.5; M26 8.5,5.5; M27 9.5,5.5; M28 10.5,5.5; M29 11.5,5.5; M30 12.5,5.5; M31 13.5,5.5; M32 14.5,5.5; M33 15.5,5.5; M34 16.5,5.5; N1 -16.5,4.5; N2 -15.5,4.5; N3 -14.5,4.5; N4 -13.5,4.5; N5 -12.5,4.5; N6 -11.5,4.5; N7 -10.5,4.5; N8 -9.5,4.5; N9 -8.5,4.5; N10 -7.5,4.5; N11 -6.5,4.5; N12 -5.5,4.5; N13 -4.5,4.5; N14 -3.5,4.5; N15 -2.5,4.5; N16 -1.5,4.5; N17 -0.5,4.5; N18 0.5,4.5; N19 1.5,4.5; N20 2.5,4.5; N21 3.5,4.5; N22 4.5,4.5; N23 5.5,4.5; N24 6.5,4.5; N25 7.5,4.5; N26 8.5,4.5; N27 9.5,4.5; N28 10.5,4.5; N29 11.5,4.5; N30 12.5,4.5; N31 13.5,4.5; N32 14.5,4.5; N33 15.5,4.5; N34 16.5,4.5; P1 -16.5,3.5; P2 -15.5,3.5; P3 -14.5,3.5; P4 -13.5,3.5; P5 -12.5,3.5; P6 -11.5,3.5; P7 -10.5,3.5; P8 -9.5,3.5; P9 -8.5,3.5; P10 -7.5,3.5; P11 -6.5,3.5; P12 -5.5,3.5; P13 -4.5,3.5; P14 -3.5,3.5; P15 -2.5,3.5; P16 -1.5,3.5; P17 -0.5,3.5; P18 0.5,3.5; P19 1.5,3.5; P20 2.5,3.5; P21 3.5,3.5; P22 4.5,3.5; P23 5.5,3.5; P24 6.5,3.5; P25 7.5,3.5; P26 8.5,3.5; P27 9.5,3.5; P28 10.5,3.5; P29 11.5,3.5; P30 12.5,3.5; P31 13.5,3.5; P32 14.5,3.5; P33 15.5,3.5; P34 16.5,3.5; R1 -16.5,2.5; R2 -15.5,2.5; R3 -14.5,2.5; R4 -13.5,2.5; R5 -12.5,2.5; R6 -11.5,2.5; R7 -10.5,2.5; R8 -9.5,2.5; R9 -8.5,2.5; R10 -7.5,2.5; R11 -6.5,2.5; R12 -5.5,2.5; R13 -4.5,2.5; R14 -3.5,2.5; R15 -2.5,2.5; R16 -1.5,2.5; R17 -0.5,2.5; R18 0.5,2.5; R19 1.5,2.5; R20 2.5,2.5; R21 3.5,2.5; R22 4.5,2.5; R23 5.5,2.5; R24 6.5,2.5; R25 7.5,2.5; R26 8.5,2.5; R27 9.5,2.5; R28 10.5,2.5; R29 11.5,2.5; R30 12.5,2.5; R31 13.5,2.5; R32 14.5,2.5; R33 15.5,2.5; R34 16.5,2.5; T1 -16.5,1.5; T2 -15.5,1.5; T3 -14.5,1.5; T4 -13.5,1.5; T5 -12.5,1.5; T6 -11.5,1.5; T7 -10.5,1.5; T8 -9.5,1.5; T9 -8.5,1.5; T10 -7.5,1.5; T11 -6.5,1.5; T12 -5.5,1.5; T13 -4.5,1.5; T14 -3.5,1.5; T15 -2.5,1.5; T16 -1.5,1.5; T17 -0.5,1.5; T18 0.5,1.5; T19 1.5,1.5; T20 2.5,1.5; T21 3.5,1.5; T22 4.5,1.5; T23 5.5,1.5; T24 6.5,1.5; T25 7.5,1.5; T26 8.5,1.5; T27 9.5,1.5; T28 10.5,1.5; T29 11.5,1.5; T30 12.5,1.5; T31 13.5,1.5; T32 14.5,1.5; T33 15.5,1.5; T34 16.5,1.5; U1 -16.5,0.5; U2 -15.5,0.5; U3 -14.5,0.5; U4 -13.5,0.5; U5 -12.5,0.5; U6 -11.5,0.5; U7 -10.5,0.5; U8 -9.5,0.5; U9 -8.5,0.5; U10 -7.5,0.5; U11 -6.5,0.5; U12 -5.5,0.5; U13 -4.5,0.5; U14 -3.5,0.5; U15 -2.5,0.5; U16 -1.5,0.5; U17 -0.5,0.5; U18 0.5,0.5; U19 1.5,0.5; U20 2.5,0.5; U21 3.5,0.5; U22 4.5,0.5; U23 5.5,0.5; U24 6.5,0.5; U25 7.5,0.5; U26 8.5,0.5; U27 9.5,0.5; U28 10.5,0.5; U29 11.5,0.5; U30 12.5,0.5; U31 13.5,0.5; U32 14.5,0.5; U33 15.5,0.5; U34 16.5,0.5; V1 -16.5,-0.5; V2 -15.5,-0.5; V3 -14.5,-0.5; V4 -13.5,-0.5; V5 -12.5,-0.5; V6 -11.5,-0.5; V7 -10.5,-0.5; V8 -9.5,-0.5; V9 -8.5,-0.5; V10 -7.5,-0.5; V11 -6.5,-0.5; V12 -5.5,-0.5; V13 -4.5,-0.5; V14 -3.5,-0.5; V15 -2.5,-0.5; V16 -1.5,-0.5; V17 -0.5,-0.5; V18 0.5,-0.5; V19 1.5,-0.5; V20 2.5,-0.5; V21 3.5,-0.5; V22 4.5,-0.5; V23 5.5,-0.5; V24 6.5,-0.5; V25 7.5,-0.5; V26 8.5,-0.5; V27 9.5,-0.5; V28 10.5,-0.5; V29 11.5,-0.5; V30 12.5,-0.5; V31 13.5,-0.5; V32 14.5,-0.5; V33 15.5,-0.5; V34 16.5,-0.5; W1 -16.5,-1.5; W2 -15.5,-1.5; W3 -14.5,-1.5; W4 -13.5,-1.5; W5 -12.5,-1.5; W6 -11.5,-1.5; W7 -10.5,-1.5; W8 -9.5,-1.5; W9 -8.5,-1.5; W10 -7.5,-1.5; W11 -6.5,-1.5; W12 -5.5,-1.5; W13 -4.5,-1.5; W14 -3.5,-1.5; W15 -2.5,-1.5; W16 -1.5,-1.5; W17 -0.5,-1.5; W18 0.5,-1.5; W19 1.5,-1.5; W20 2.5,-1.5; W21 3.5,-1.5; W22 4.5,-1.5; W23 5.5,-1.5; W24 6.5,-1.5; W25 7.5,-1.5; W26 8.5,-1.5; W27 9.5,-1.5; W28 10.5,-1.5; W29 11.5,-1.5; W30 12.5,-1.5; W31 13.5,-1.5; W32 14.5,-1.5; W33 15.5,-1.5; W34 16.5,-1.5; Y1 -16.5,-2.5; Y2 -15.5,-2.5; Y3 -14.5,-2.5; Y4 -13.5,-2.5; Y5 -12.5,-2.5; Y6 -11.5,-2.5; Y7 -10.5,-2.5; Y8 -9.5,-2.5; Y9 -8.5,-2.5; Y10 -7.5,-2.5; Y11 -6.5,-2.5; Y12 -5.5,-2.5; Y13 -4.5,-2.5; Y14 -3.5,-2.5; Y15 -2.5,-2.5; Y16 -1.5,-2.5; Y17 -0.5,-2.5; Y18 0.5,-2.5; Y19 1.5,-2.5; Y20 2.5,-2.5; Y21 3.5,-2.5; Y22 4.5,-2.5; Y23 5.5,-2.5; Y24 6.5,-2.5; Y25 7.5,-2.5; Y26 8.5,-2.5; Y27 9.5,-2.5; Y28 10.5,-2.5; Y29 11.5,-2.5; Y30 12.5,-2.5; Y31 13.5,-2.5; Y32 14.5,-2.5; Y33 15.5,-2.5; Y34 16.5,-2.5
